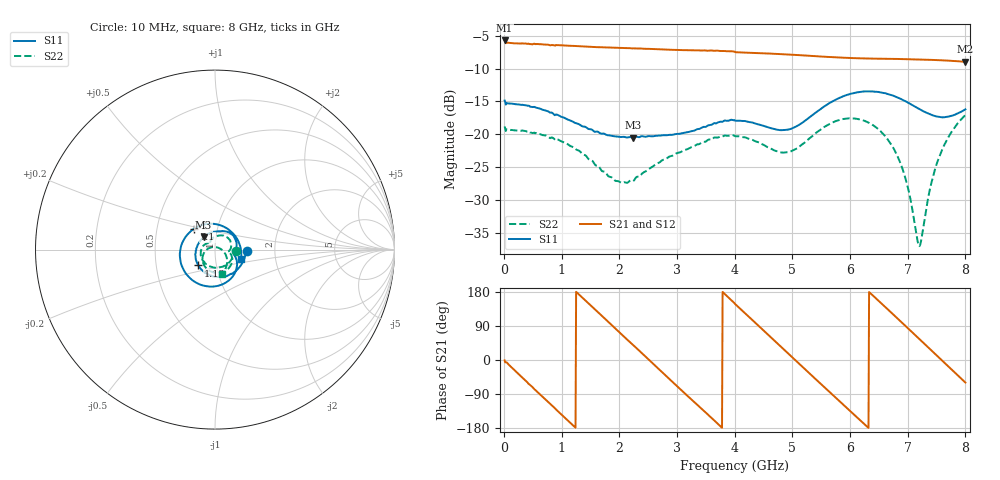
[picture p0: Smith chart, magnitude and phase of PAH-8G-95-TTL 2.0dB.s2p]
! MTS Systemtechnik GmbH
! S-Parameters
! Model: PAH-8G/95-TTL
! Attenuation Step: 2.0dB
! Rohde & Schwarz ZVB8 2Ports - Version 4.11 - 1145.1010k08 SN: 100119
! S2P File Measurements:
! S11 S21 S12 S22
# HZ  S  DB  R  50.00
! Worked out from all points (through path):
!   800 points, 10 MHz to 8 GHz, reference 50 ohm
!   highest |S21| = -5.72 dB at 10 MHz (marker M1); lowest = -9.0 dB at 8 GHz (marker M2)
!   group delay of S21, straight-line fit = 395 ps
!   lowest |S11| = -20.5 dB at 2.24 GHz (marker M3), VSWR 1.21, Z = 43.6 + j6.07 ohm
!   |S11| at or under -10 dB: start of sweep to end of sweep
!   |S22| runs from -37.1 to -17.1 dB; largest |S21 - S12| = 0.0063
!   S11 on the Smith chart (normalised r, x): 10 MHz: 1.44, -0.02; 1.13 GHz: 0.82, -0.15; 7.1 GHz: 0.77, +0.18; 8 GHz: 1.33, -0.15
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1e7  -14.87 -1.9  -5.72 -1.1  -5.65 -1.0  -18.82 -2.6
5.9e8  -16.03 -74.0  -6.26 -86.1  -6.27 -86.1  -19.89 -89.5
1.13e9  -17.86 -136.5  -6.53 -163.0  -6.53 -163.1  -21.70 -164.7
1.35e9  -18.77 -159.2  -6.62 165.6  -6.62 165.6  -22.93 168.6
1.81e9  -20.17 162.3  -6.79 100.1  -6.80 100.3  -26.40 131.7
2.24e9  -20.52 132.8  -6.92 39.5  -6.91 39.4  -27.14 124.9
2.68e9  -20.23 105.8  -7.07 -23.5  -7.06 -23.3  -24.37 109.4
2.99e9  -19.96 88.5  -7.16 -67.7  -7.15 -67.9  -22.91 92.0
3.27e9  -19.51 74.8  -7.23 -107.1  -7.25 -107.5  -21.91 75.5
3.67e9  -18.36 53.2  -7.27 -163.2  -7.25 -162.8  -20.50 50.9
4.01e9  -17.95 29.6  -7.51 147.3  -7.51 147.2  -20.32 26.8
4.55e9  -18.87 -2.7  -7.70 70.6  -7.72 70.6  -21.88 -4.0
4.95e9  -19.25 -14.2  -7.87 13.5  -7.87 13.5  -22.70 -9.5
5.34e9  -17.16 -28.6  -8.08 -41.6  -8.08 -41.6  -20.34 -18.8
5.72e9  -14.88 -57.5  -8.28 -94.9  -8.30 -95.0  -18.12 -45.4
6.13e9  -13.62 -99.6  -8.43 -152.7  -8.44 -152.7  -17.68 -83.9
6.67e9  -13.93 -164.3  -8.51 131.3  -8.52 131.4  -21.01 -141.5
6.92e9  -14.81 162.0  -8.56 95.7  -8.56 95.7  -25.55 -173.2
7.1e9  -15.66 135.4  -8.59 70.0  -8.59 70.0  -32.56 147.4
7.22e9  -16.25 116.2  -8.62 52.7  -8.61 52.8  -36.74 67.6
7.52e9  -17.32 63.6  -8.71 9.7  -8.71 9.6  -24.07 -22.9
8e9  -16.21 -20.1  -8.97 -59.5  -8.97 -59.6  -17.07 -73.2
